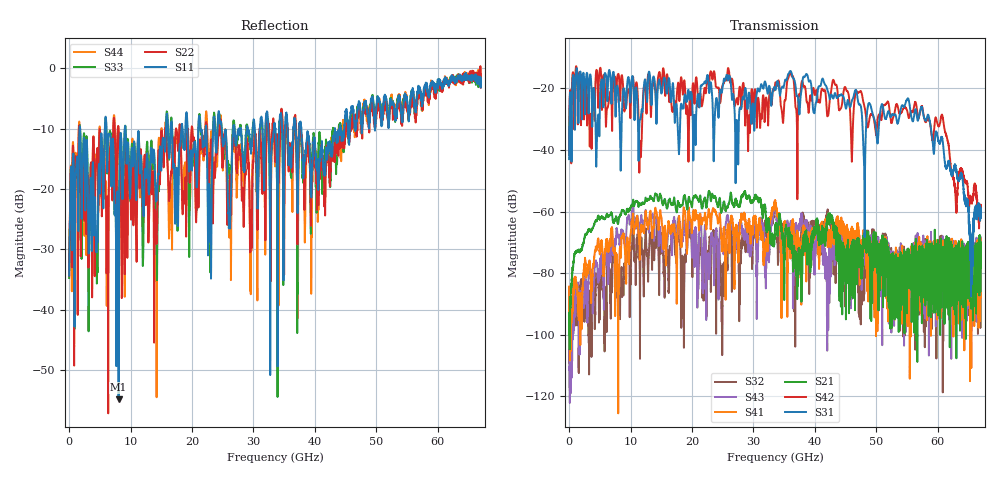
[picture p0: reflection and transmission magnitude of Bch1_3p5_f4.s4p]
!Agilent Technologies,N5247A,US51170199,A.09.90.13
!Agilent N5247A: A.09.90.13
!Date: Thursday, October 18, 2018 11:21:37
!Correction: S11(Full 4 Port(1,2,3,4))
!S12(Full 4 Port(1,2,3,4))
!S13(Full 4 Port(1,2,3,4))
!S14(Full 4 Port(1,2,3,4))
!S21(Full 4 Port(1,2,3,4))
!S22(Full 4 Port(1,2,3,4))
!S23(Full 4 Port(1,2,3,4))
!S24(Full 4 Port(1,2,3,4))
!S31(Full 4 Port(1,2,3,4))
!S32(Full 4 Port(1,2,3,4))
!S33(Full 4 Port(1,2,3,4))
!S34(Full 4 Port(1,2,3,4))
!S41(Full 4 Port(1,2,3,4))
!S42(Full 4 Port(1,2,3,4))
!S43(Full 4 Port(1,2,3,4))
!S44(Full 4 Port(1,2,3,4))
!S4P File: Measurements: <S11,S12,S13,S14>,
!<S21,S22,S23,S24>,
!<S31,S32,S33,S34>,
!<S41,S42,S43,S44>:
# Hz S  dB  R 50
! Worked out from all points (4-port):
!   6701 points, 10 MHz to 67 GHz, reference 50 ohm
!   strongest paths, dB at 10 MHz, 16.76 GHz, 33.51 GHz, 50.25 GHz, 67 GHz:
!     S31: -43.0, -20.9, -20.2, -36.9, -60.6
!     S42: -41.6, -27.5, -18.9, -29.5, -58.2
!     S21: -95.8, -57.5, -65.1, -73.4, -76.9
!     S41: -84.4, -64.3, -57.1, -83.5, -88.0
!     S43: -91.4, -73.0, -57.1, -77.6, -78.6
!     S32: -84.6, -68.7, -57.9, -71.0, -75.7
!   lowest |S11| = -54.9 dB at 8.059 GHz (marker M1), VSWR 1.00, Z = 50.1 + j0.111 ohm
!   |S11| at or under -10 dB: 1.794 GHz to 5.823 GHz (4.029 GHz wide, 106 % of centre); 9.191 GHz to 15.77 GHz (6.582 GHz wide, 52.7 % of centre); 37.81 GHz to 43.24 GHz (5.433 GHz wide, 13.4 % of centre)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
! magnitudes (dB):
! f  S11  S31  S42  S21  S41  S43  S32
! 10 MHz  -34.4  -43.0  -41.6  -95.8  -84.4  -91.4  -84.6
! 8.059 GHz  -54.9  -22.7  -15.4  -63.2  -86.2  -67.8  -82.7
! 11.61 GHz  -15.2  -30.0  -39.8  -57.9  -67.2  -63.9  -76.4
! 14.65 GHz  -15.9  -17.2  -14.9  -56.1  -64.5  -69.8  -86.4
! 33.4 GHz  -9.6  -19.6  -20.7  -68.1  -57.4  -57.8  -58.9
! 55.06 GHz  -6.1  -23.4  -27.7  -77.3  -83.5  -76.5  -84.6
! 67 GHz  -3.2  -60.6  -58.2  -76.9  -88.0  -78.6  -75.7
